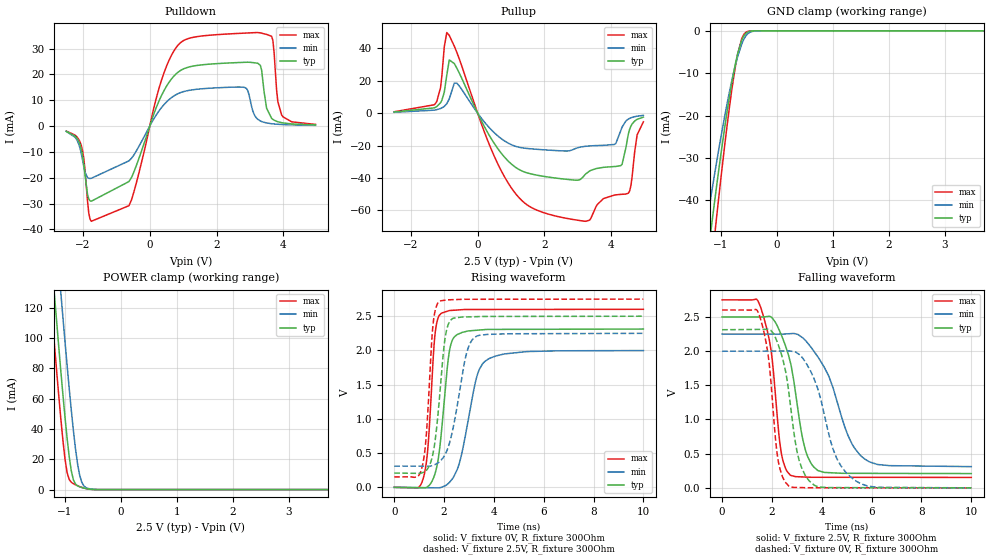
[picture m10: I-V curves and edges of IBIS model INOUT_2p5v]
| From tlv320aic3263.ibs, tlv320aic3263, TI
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|   INOUT_2p5v
[Model]   INOUT_2p5v
Model_type   I/O
Polarity   Non-Inverting
Enable   Active-High
Vinl = 0.75
Vinh = 1.75
Vmeas = 1.25
Vref = 0
Cref = 5pF
Rref = 10000
|   typ   min   max
C_comp   1.460pF   1.439pF   1.501pF
[Voltage Range]   2.5   2.25   2.75
[Temperature Range]   27   125   -40
[Pullup Reference]   2.5   2.25   2.75
[Pulldown Reference]   -0   -0   -0
[Power Clamp Reference]   2.5   2.25   2.75
[GND Clamp Reference]   -0   -0   -0
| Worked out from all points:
|   slope of the pulldown table from 0 to 0.375 V, typ, clamps not added: 30.2 ohm
|   slope of the pullup table from 0 to 0.375 V, typ, clamps not added: 25.6 ohm
|   GND clamp passes 1 mA (typ) near -0.58 V on its own axis
|   POWER clamp passes 1 mA (typ) near -0.66 V on its own axis
|   falling waveform, V_fixture 2.5V, R_fixture 300Ohm: 20-80 % time 689ps typ, 1.2ns min, 458ps max; typ from 2.5 V to 0.209 V
|   rising waveform, V_fixture 0V, R_fixture 300Ohm: 20-80 % time 376ps typ, 653ps min, 262ps max; typ from 0 V to 2.31 V
|   rising waveform, V_fixture 2.5V, R_fixture 300Ohm: 20-80 % time 358ps typ, 584ps min, 256ps max; typ from 0.209 V to 2.5 V
|   falling waveform, V_fixture 0V, R_fixture 300Ohm: 20-80 % time 594ps typ, 959ps min, 414ps max; typ from 2.31 V to 0 V
[Pulldown]
|   Voltage   I(typ)   I(min)   I(max)
-2.5V     -2.047mA   -2.081mA   -1.931mA
-2.05V    -8.946mA   -10.67mA   -7.569mA
-1.75V    -29.09mA   -20.22mA   -36.88mA
-625mV    -21.5mA    -13.48mA   -30.84mA
312.5mV   10.77mA    6.509mA    16.16mA
800mV     20.34mA    12.26mA    30.59mA
2.825V    24.69mA    15mA       35.99mA
3.2V      24.41mA    3.073mA    36.22mA
3.65V     2.994mA    918.5uA    34.78mA
3.837V    1.675mA    701.3uA    9.361mA
3.95V     1.316mA    613.5uA    4.304mA
4.963V    439.8uA    285.8uA    649.2uA
[GND Clamp]
|   Voltage   I(typ)   I(min)   I(max)
-2.5V     -396.4mA   -332.1mA   -445.5mA
-1.3V     -60.4mA    -49.49mA   -72.67mA
-1.225V   -52.22mA   -43.11mA   -62.86mA
-1.188V   -48.21mA   -39.98mA   -58.02mA
-1.113V   -40.39mA   -33.88mA   -48.54mA
-1.075V   -36.58mA   -30.91mA   -43.9mA
-887.5mV  -19mA      -17.13mA   -22.28mA
-737.5mV  -7.645mA   -7.979mA   -8.22mA
-625mV    -2.148mA   -3.053mA   -1.781mA
-550mV    -539.7uA   -1.149mA   -311uA
-325mV    -899.8nA   -11.65uA   -63.22nA
4.963V    0A         0A         0A
[Pullup]
|   Voltage   I(typ)   I(min)   I(max)
-2.5V     767.5uA    573.1uA    910.9uA
-1.262V   3.678mA    2.042mA    6.088mA
-1.113V   6.468mA    2.919mA    15.74mA
-925mV    23.54mA    5.867mA    49.8mA
-850mV    32.88mA    8.905mA    48.04mA
-625mV    27.84mA    18.6mA     37.6mA
1.062V    -32.27mA   -19.88mA   -47.66mA
3.237V    -37.44mA   -20.4mA    -66.71mA
4.287V    -32.33mA   -10.64mA   -50.08mA
4.55V     -10mA      -3.182mA   -48.07mA
4.775V    -3.778mA   -1.821mA   -13.39mA
4.963V    -2.398mA   -1.326mA   -5.289mA
[POWER Clamp]
|   Voltage   I(typ)   I(min)   I(max)
-2.5V     760.7mA    810.8mA    730.1mA
-1.262V   162.2mA    215mA      129.3mA
-1.188V   127.9mA    180.6mA    95.07mA
-1.075V   78.32mA    130mA      46.81mA
-1V       47.7mA     97.58mA    20.16mA
-962.5mV  33.86mA    81.91mA    11.22mA
-887.5mV  12.32mA    52.35mA    4.821mA
-775mV    2.459mA    16.85mA    2.546mA
-737.5mV  1.825mA    9.412mA    1.979mA
-662.5mV  1.016mA    2.426mA    1.034mA
-475mV    68.02uA    163.6uA    31.07uA
4.963V    0A         0A         0A
[Ramp]
R_load = 300
|   typ   min   max
dV/dt_r   1.38785/3.7469e-010   1.19892/6.51106e-010   1.56086/2.62167e-010
dV/dt_f   1.37466/6.82954e-010   1.16375/1.19462e-009   1.55843/4.55603e-010
[Falling Waveform]
V_fixture = 2.5V
V_fixture_min = 2.25V
V_fixture_max = 2.75V
R_fixture = 300Ohm
C_fixture = 0F
|   Time   V(typ)   V(min)   V(max)
0s        2.5V       2.25V      2.75V
1.506ns   2.499V     2.25V      2.681V
1.964ns   2.5V       2.25V      2.013V
2.369ns   2.244V     2.249V     525.4mV
2.739ns   1.837V     2.256V     185.7mV
3.333ns   565.1mV    2.16V      158.2mV
3.831ns   257.1mV    1.923V     154.8mV
5.054ns   212.6mV    763.5mV    154.3mV
5.721ns   212.1mV    422.5mV    154.1mV
10ns      208.9mV    310.4mV    152.6mV
[Rising Waveform]
V_fixture = 0V
V_fixture_min = 0V
V_fixture_max = 0V
R_fixture = 300Ohm
C_fixture = 0F
|   Time   V(typ)   V(min)   V(max)
0s        628.3nV    773.1nV    331.7nV
1.175ns   -5.425mV   -4.912mV   142.6mV
1.368ns   17.32mV    -5.718mV   650.5mV
1.65ns    214.7mV    -6.895mV   2.271V
1.885ns   774.5mV    -409.6uV   2.541V
2.161ns   1.848V     53.81mV    2.577V
2.334ns   2.152V     124.7mV    2.586V
3.306ns   2.295V     1.606V     2.598V
3.658ns   2.305V     1.846V     2.599V
10ns      2.313V     1.998V     2.601V
[Rising Waveform]
V_fixture = 2.5V
V_fixture_min = 2.25V
V_fixture_max = 2.75V
R_fixture = 300Ohm
C_fixture = 0F
|   Time   V(typ)   V(min)   V(max)
0s        208.9mV    310mV      152.6mV
1.112ns   211.7mV    309.4mV    286.4mV
1.295ns   252.5mV    309.3mV    796.1mV
1.554ns   490.1mV    320.5mV    2.363V
1.806ns   1.262V     371mV      2.717V
2.02ns    2.124V     466.5mV    2.734V
2.199ns   2.405V     622.5mV    2.74V
2.903ns   2.49V      1.958V     2.748V
3.306ns   2.494V     2.209V     2.748V
10ns      2.5V       2.25V      2.75V
[Falling Waveform]
|Gnd
V_fixture = 0V
V_fixture_min = 0V
V_fixture_max = 0V
R_fixture = 300Ohm
C_fixture = 0F
|   Time   V(typ)   V(min)   V(max)
0s        2.313V     1.998V     2.601V
1.482ns   2.318V     2V         2.539V
1.868ns   2.318V     2.001V     1.883V
2.246ns   2.101V     2.001V     406.7mV
2.676ns   1.403V     2.002V     27.02mV
3.085ns   410.5mV    1.954V     4.923mV
3.723ns   34.62mV    1.564V     1.679mV
4.584ns   3.82mV     445.5mV    1.449mV
5.405ns   3.241mV    92.93mV    1.229mV
10ns      2.596uV    168.6uV    80.73nV
